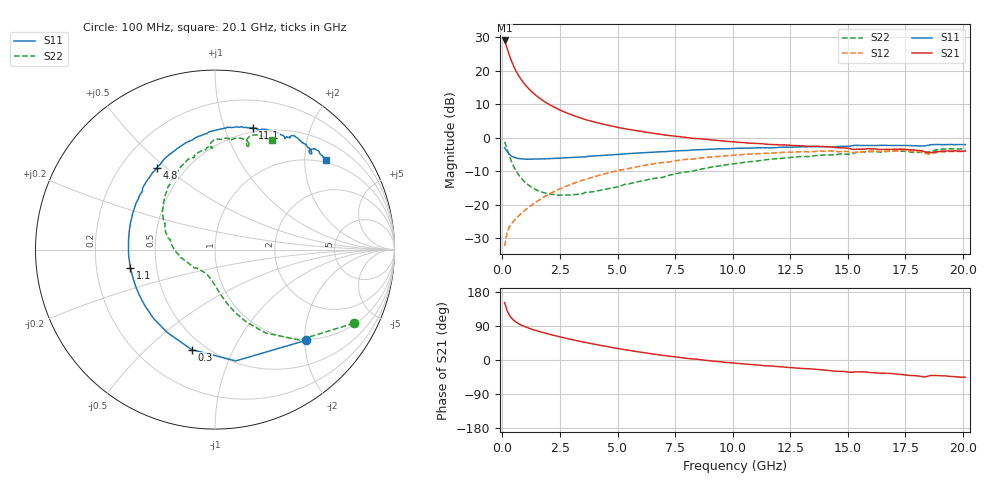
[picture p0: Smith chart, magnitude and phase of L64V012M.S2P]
!  Infineon Technologies AG
! BFR380L3 , PF131585-7, No.6, Th 09.10.01, soldered on pcb-board, measured with PP GSG850
!  Vce=4.0 V,  Ic=12.5 mA
! Common Emitter S-Parameters:  15. November 2001
#  GHz  S  MA  R  50
! f  S11  S21  S12  S22
! GHz  Mag  Ang  Mag  Ang  Mag  Ang  Mag  Ang
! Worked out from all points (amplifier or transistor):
!   201 points, 100 MHz to 20.1 GHz, reference 50 ohm
!   highest |S21| = 29.1 dB at 100 MHz (marker M1)
!   |S21| within 3 dB of that: start of sweep to 239.6 MHz
!   unconditionally stable (mu >= 1): 1.713 GHz to 4.42 GHz
!   at 3.4 GHz: K = 1.03, MAG = 8.4 dB, |S12| = -12.8 dB
!   at 10.1 GHz: K = 0.95, MSG = 2.0 dB, |S12| = -5.1 dB
!   at 20.1 GHz: K = 0.99, MSG = 0.1 dB, |S12| = -4.0 dB
!   S11 on the Smith chart (normalised r, x): 100 MHz: 0.97, -2.02; 300 MHz: 0.42, -0.70; 1.1 GHz: 0.35, -0.09; 4.8 GHz: 0.35, +0.47; 11.1 GHz: 0.46, +1.25; 20.1 GHz: 0.93, +2.53
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0.1  0.7147 -45.1  28.41 151.3  0.0242 69.5  0.8753 -27.9
0.2  0.6308 -79.4  22.17 131.4  0.03772 58.2  0.6895 -47.0
0.3  0.5722 -103.1  17.33 119.0  0.04679 52.6  0.5432 -58.8
0.4  0.5333 -119.8  13.97 110.6  0.05262 50.9  0.4413 -66.5
0.5  0.5144 -131.7  11.59 104.6  0.05782 51.2  0.3713 -72.0
0.6  0.5005 -141.0  9.874 100.0  0.06323 51.8  0.3212 -76.1
0.7  0.4923 -148.7  8.597 96.1  0.06826 52.8  0.2836 -79.6
0.8  0.4877 -154.6  7.592 92.9  0.0735 54.0  0.2552 -82.5
0.9  0.4844 -159.6  6.799 90.1  0.07871 54.8  0.2329 -85.0
1.1  0.4824 -168.0  5.633 85.2  0.08988 56.6  0.2018 -89.7
1.3  0.4818 -174.9  4.805 80.9  0.1011 57.9  0.1804 -93.9
1.5  0.482 179.4  4.196 77.1  0.1126 58.6  0.1657 -97.9
2  0.4888 167.7  3.199 68.6  0.1428 59.1  0.1465 -107.8
2.6  0.5008 156.5  2.512 59.7  0.1792 58.1  0.1402 -120.0
3.5  0.5184 142.0  1.924 47.6  0.2349 54.6  0.1473 -136.1
4.8  0.5592 125.4  1.488 32.5  0.3121 47.7  0.1802 -161.1
6.8  0.6191 104.1  1.138 13.5  0.4215 34.9  0.2545 168.3
10.1  0.6942 79.0  0.8669 -8.3  0.5532 13.4  0.4134 131.8
11.1  0.7112 72.8  0.8232 -13.5  0.5824 6.8  0.4543 122.2
13.5  0.7382 60.8  0.7486 -24.1  0.6266 -7.9  0.5381 102.0
16.8  0.7709 48.4  0.6765 -35.3  0.6346 -24.3  0.6307 79.5
20.1  0.7952 38.9  0.6376 -45.6  0.6275 -38.3  0.6882 62.7
